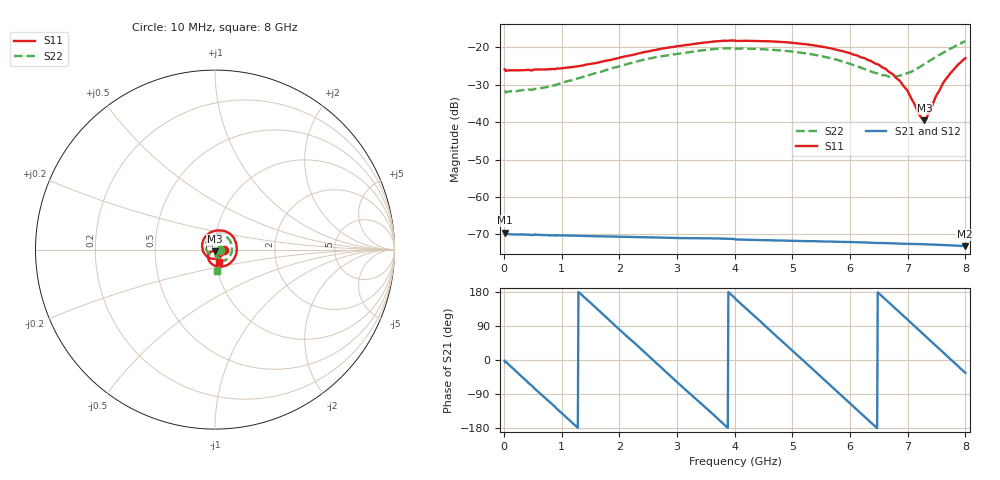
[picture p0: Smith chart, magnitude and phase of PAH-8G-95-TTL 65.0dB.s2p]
! MTS Systemtechnik GmbH
! S-Parameters
! Model: PAH-8G/95-TTL
! Attenuation Step: 65.0dB
! Rohde & Schwarz ZVB8 2Ports - Version 4.11 - 1145.1010k08 SN: 100119
! S2P File Measurements:
! S11 S21 S12 S22
# HZ  S  DB  R  50.00
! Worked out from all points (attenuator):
!   800 points, 10 MHz to 8 GHz, reference 50 ohm
!   highest |S21| = -69.51 dB at 10 MHz (marker M1); lowest = -73.2 dB at 7.99 GHz (marker M2)
!   lowest |S11| = -39.5 dB at 7.29 GHz (marker M3), VSWR 1.02, Z = 49.8 - j1.04 ohm
!   |S11| at or under -10 dB: start of sweep to end of sweep
!   |S22| runs from -32.1 to -18.4 dB; largest |S21 - S12| = 5.3e-06
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1e7  -25.88 -2.5  -69.51 -1.7  -69.46 -1.4  -31.63 -4.5
7.7e8  -25.81 -74.3  -70.20 -108.1  -70.18 -108.2  -30.55 -88.3
1.35e9  -24.89 -131.8  -70.40 171.3  -70.41 171.3  -27.99 -147.9
2.05e9  -22.59 165.3  -70.62 73.6  -70.64 73.8  -24.80 152.6
2.68e9  -20.53 116.5  -70.86 -13.8  -70.86 -13.5  -22.54 108.0
3.39e9  -18.88 68.2  -71.06 -111.5  -71.10 -112.0  -20.91 62.2
4.01e9  -18.28 27.3  -71.36 161.7  -71.37 161.7  -20.32 24.5
4.63e9  -18.39 -12.3  -71.60 75.8  -71.62 75.8  -20.61 -11.4
5.34e9  -19.40 -57.9  -71.80 -22.4  -71.81 -22.4  -21.87 -49.7
6.11e9  -22.09 -108.1  -72.11 -129.8  -72.13 -129.7  -24.98 -81.2
6.49e9  -24.61 -132.2  -72.30 177.3  -72.31 177.2  -27.06 -84.1
6.67e9  -26.51 -141.8  -72.39 152.1  -72.39 152.2  -27.85 -80.2
6.85e9  -28.77 -150.4  -72.47 127.2  -72.49 127.0  -27.59 -74.1
6.97e9  -31.08 -152.7  -72.54 110.4  -72.56 110.4  -27.04 -70.2
7.21e9  -38.24 -130.9  -72.60 76.7  -72.63 76.8  -25.23 -65.4
7.29e9  -39.51 -100.2  -72.65 65.4  -72.66 65.4  -24.45 -65.2
7.34e9  -38.43 -83.1  -72.69 58.3  -72.71 58.4  -23.95 -65.4
7.49e9  -33.06 -59.0  -72.77 37.3  -72.78 37.4  -22.52 -67.6
7.64e9  -28.94 -57.9  -72.87 16.5  -72.88 16.4  -21.24 -71.7
7.84e9  -25.15 -65.5  -73.02 -11.6  -73.03 -11.6  -19.53 -79.0
7.99e9  -22.98 -72.6  -73.16 -32.4  -73.15 -32.4  -18.43 -85.2
8e9  -22.86 -73.2  -73.15 -33.8  -73.15 -33.7  -18.37 -85.8
